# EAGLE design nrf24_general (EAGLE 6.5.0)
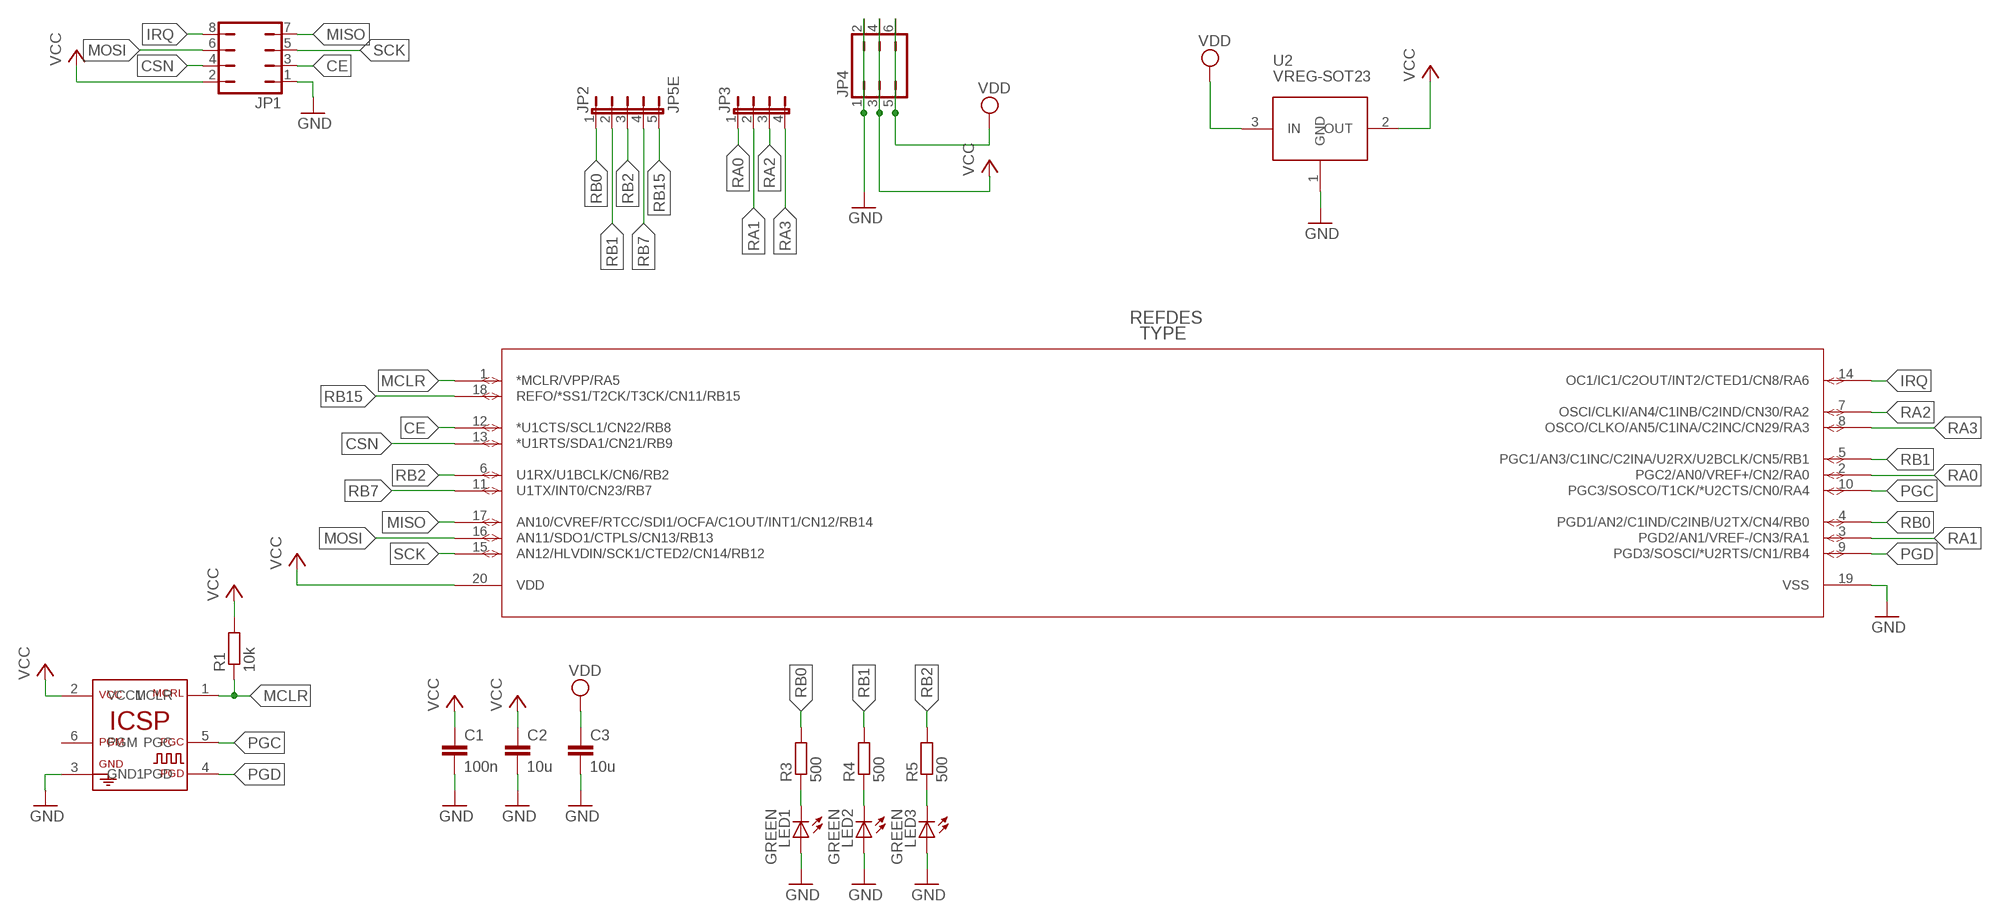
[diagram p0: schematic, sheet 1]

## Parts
C1  100n  C-EUC0603  [C0603]
C2  10u  C-EUC0805  [C0805]
C3  10u  C-EUC0805  [C0805]
ICSP  PICKIT3  [PICKIT3]
JP1  JP4Q  [JP4Q]
JP2  JP5E  [JP5]
JP3  JP4E  [JP4]
JP4  JP3Q  [JP3Q]
LED1  GREEN  LEDCHIP-LED0603  [CHIP-LED0603]
LED2  GREEN  LEDCHIP-LED0603  [CHIP-LED0603]
LED3  GREEN  LEDCHIP-LED0603  [CHIP-LED0603]
R1  10k  R-EU_R0603  [R0603]
R3  500  R-EU_R0603  [R0603]
R4  500  R-EU_R0603  [R0603]
R5  500  R-EU_R0603  [R0603]
U2  VREG-SOT23  [SOT-23]
U3  PIC24F16KA101-X_  [SSOP20_MC]

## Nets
CE: JP1.3 U3.12(*U1CTS/SCL1/CN22/RB8)
CSN: JP1.4 U3.13(*U1RTS/SDA1/CN21/RB9)
GND: C1.2 C2.2 C3.2 ICSP.3(GND1) JP1.1 JP4.1 JP4.2 LED1.A LED2.A LED3.A U2.1(GND) U3.19(VSS)
IRQ: JP1.8 U3.14(OC1/IC1/C2OUT/INT2/CTED1/CN8/RA6)
MCLR: ICSP.1(MCLR) R1.1 U3.1(*MCLR/VPP/RA5)
MISO: JP1.7 U3.17(AN10/CVREF/RTCC/SDI1/OCFA/C1OUT/INT1/CN12/RB14)
MOSI: JP1.6 U3.16(AN11/SDO1/CTPLS/CN13/RB13)
N$2: LED1.C R3.1
N$3: LED2.C R4.1
N$4: LED3.C R5.1
PGC: ICSP.5(PGC) U3.10(PGC3/SOSCO/T1CK/*U2CTS/CN0/RA4)
PGD: ICSP.4(PGD) U3.9(PGD3/SOSCI/*U2RTS/CN1/RB4)
RA0: JP3.1 U3.2(PGC2/AN0/VREF+/CN2/RA0)
RA1: JP3.2 U3.3(PGD2/AN1/VREF-/CN3/RA1)
RA2: JP3.3 U3.7(OSCI/CLKI/AN4/C1INB/C2IND/CN30/RA2)
RA3: JP3.4 U3.8(OSCO/CLKO/AN5/C1INA/C2INC/CN29/RA3)
RB0: JP2.1 R3.2 U3.4(PGD1/AN2/C1IND/C2INB/U2TX/CN4/RB0)
RB1: JP2.2 R4.2 U3.5(PGC1/AN3/C1INC/C2INA/U2RX/U2BCLK/CN5/RB1)
RB2: JP2.3 R5.2 U3.6(U1RX/U1BCLK/CN6/RB2)
RB7: JP2.4 U3.11(U1TX/INT0/CN23/RB7)
RB15: JP2.5 U3.18(REFO/*SS1/T2CK/T3CK/CN11/RB15)
SCK: JP1.5 U3.15(AN12/HLVDIN/SCK1/CTED2/CN14/RB12)
VCC: C1.1 C2.1 ICSP.2(VCC1) JP1.2 JP4.3 JP4.4 R1.2 U2.2(OUT) U3.20(VDD)
VDD: C3.1 JP4.5 JP4.6 U2.3(IN)

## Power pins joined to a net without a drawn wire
PGM: ICSP.6(PGM)

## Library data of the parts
C1-C3 = rcl:C-EU: CAPACITOR, European symbol
ICSP = other:PICKIT3
JP1 = jumper_own:JP4Q: JUMPER
JP2 = jumper_own:JP5E
JP3 = jumper_own:JP4E: JUMPER
JP4 = jumper:JP3Q: JUMPER
LED1-LED3 = led:LED: LED
R1 R3-R5 = rcl:R-EU_: RESISTOR, European symbol
U2 = other:VREG-SOT23
U3 = microchip:PIC24F16KA101-X_

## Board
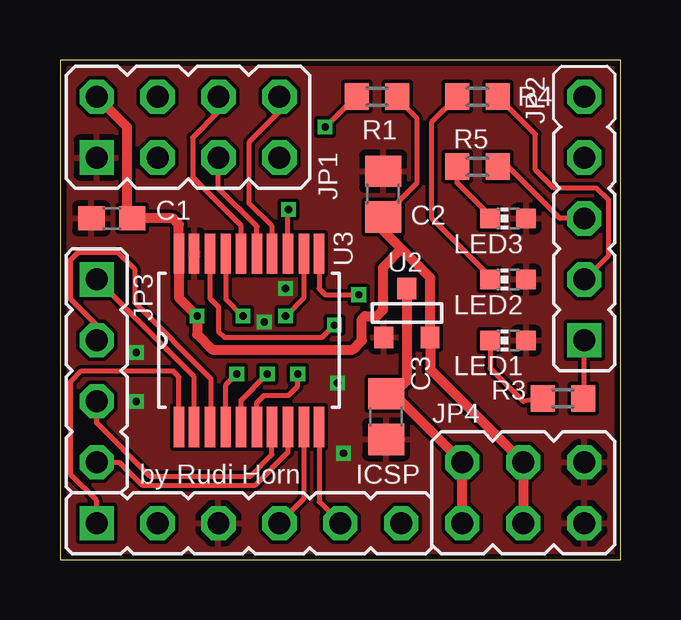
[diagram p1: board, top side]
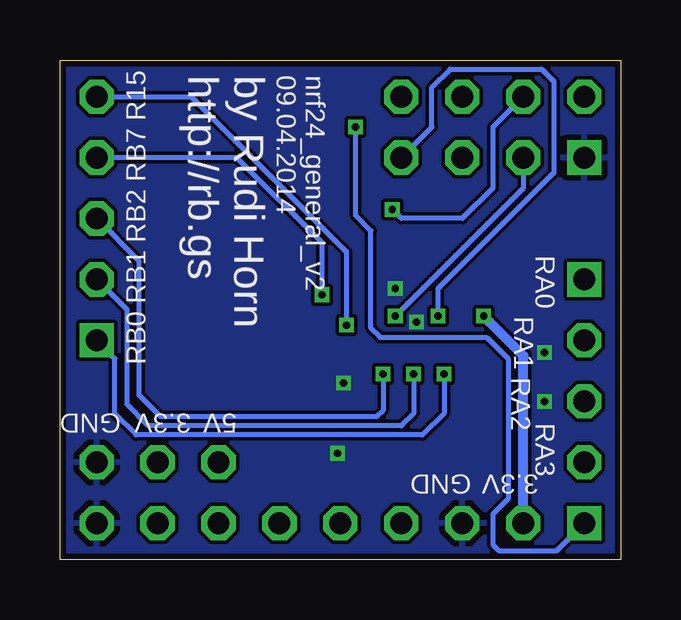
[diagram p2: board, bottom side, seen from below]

Size 23.37 x 20.83 mm. Coordinates in mm from the lower left corner, seen from the top.
Outline: 0,0 23.37,0 23.37,20.83 0,20.83 0,0
Copper layers (1*16): Top 0.035mm / dielectric 1.5mm / Bottom 0.035mm
Design rules "Elecrow_2-layer_eagle_rule": minimum track width 6mil, minimum drill 12mil, track to track 6mil, track to pad 6mil, pad to pad 6mil, via to via 6mil, smd to smd 0mil, copper to edge 10mil, drill to drill 10mil, minimum pad ring 10mil, minimum via ring 6mil, stop-mask expansion 2mil, vias tented up to drill 100mil, thermal gap 10mil

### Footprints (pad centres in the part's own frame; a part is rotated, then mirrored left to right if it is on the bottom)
C0603 = smd 1.1 x 1: 1 -0.85,0; 2 0.85,0
C0805 = smd 1.3 x 1.5: 1 -0.95,0; 2 0.95,0
PICKIT3 = drill 0.914 square: 1 -3.81,0 | drill 0.914 octagon: 2 -1.27,0; 3 1.27,0; 4 3.81,0; 5 6.35,0; 6 8.89,0
JP4Q = drill 0.914 square: 1 -3.81,-1.27 | drill 0.914 octagon: 2 -3.81,1.27; 3 -1.27,-1.27; 4 -1.27,1.27; 5 1.27,-1.27; 6 1.27,1.27; 7 3.81,-1.27; 8 3.81,1.27
JP5 = drill 0.914 square: 1 -3.81,0 | drill 0.914 octagon: 2 -1.27,0; 3 1.27,0; 4 3.81,0; 5 6.35,0
JP4 = drill 0.914 square: 1 -3.81,0 | drill 0.914 octagon: 2 -1.27,0; 3 1.27,0; 4 3.81,0
JP3Q = drill 0.914 octagon: 1 -2.54,-1.27; 2 -2.54,1.27; 3 0,-1.27; 4 0,1.27; 5 2.54,-1.27; 6 2.54,1.27
CHIP-LED0603 = smd 0.8 x 0.8: A 0,-0.75; C 0,0.75
R0603 = smd 1 x 1.1: 1 -0.85,0; 2 0.85,0
SOT-23 = smd 0.787 x 0.889: 1 0.991,1.016; 2 -0.94,1.016; 3 0.025,-1.016
SSOP20_MC = smd 1.676 x 0.432: 1 -3.607,2.921; 2 -3.607,2.286; 3 -3.607,1.626; 4 -3.607,0.965; 5 -3.607,0.33; 6 -3.607,-0.33; 7 -3.607,-0.965; 8 -3.607,-1.626; 9 -3.607,-2.286; 10 -3.607,-2.921; 11 3.607,-2.921; 12 3.607,-2.286; 13 3.607,-1.626; 14 3.607,-0.965; 15 3.607,-0.33; 16 3.607,0.33; 17 3.607,0.965; 18 3.607,1.626; 19 3.607,2.286; 20 3.607,2.921

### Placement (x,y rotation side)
C1  2.16,14.22 180 top
C2  13.46,15.24 90 top
C3  13.59,5.97 270 top
ICSP  5.33,1.52 0 top
JP1  5.33,18.03 0 top
JP2  21.84,12.95 90 top
JP3  1.52,7.87 270 top
JP4  19.3,2.79 180 top
LED1  18.67,9.14 90 top
LED2  18.67,11.68 90 top
LED3  18.67,14.22 90 top
R1  13.21,19.3 0 top
R3  20.96,6.73 0 top
R4  17.4,19.3 0 top
R5  17.4,16.38 0 top
U2  14.48,10.29 180 top
U3  7.87,9.14 90 top

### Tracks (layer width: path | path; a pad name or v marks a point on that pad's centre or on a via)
CE  (via drill 0.3 pad 0.2)
  Top 0.203: U3.12 10.16,10.92 v9.4,10.16
  Bottom 0.203: JP1.3 4.06,15.49 v9.4,10.16
CSN  (via drill 0.3)
  Top 0.203: U3.13 9.5,14.45 v9.53,14.61
  Bottom 0.203: JP1.4 5.33,18.03 5.33,15.49 6.6,14.22 9.14,14.22 v9.53,14.61
GND  (via drill 0.3)
  other vias: 3.17,6.6 3.17,8.64 9.4,11.3 8.51,9.91 11.56,7.37 11.81,4.45
  pour Top: 0,0 23.37,0 23.37,20.83 0,20.83
  pour Bottom: 23.37,0 0,0 0,20.83 23.37,20.83
IRQ
  Top 0.203: JP1.8 9.14,18.67 7.87,17.4 7.87,14.86 8.84,13.89 U3.14
MCLR  (via drill 0.3)
  Top 0.203: ICSP.1 1.52,2.48 0.45,3.56 0.45,7.43 0.89,7.87 4.7,7.87 4.95,7.62 U3.1 | R1.1 12.32,19.3 v11.05,18.03
  Bottom 0.203: ICSP.1 2.67,0.38 5.08,0.38 5.33,0.64 5.33,1.91 4.7,2.54 4.7,8.38 5.59,9.27 10.03,9.27 10.41,9.65 10.41,13.72 11.05,14.35 v11.05,18.03
MISO  (via drill 0.3)
  Top 0.203: v7.62,10.16 6.91,10.87 U3.17
  Bottom 0.203: JP1.7 7.87,18.03 7.87,19.69 7.11,20.45 3.3,20.45 2.79,19.94 2.79,16.13 7.62,11.3 v7.62,10.16
MOSI
  Top 0.203: JP1.6 6.6,18.67 5.53,17.59 5.53,15.94 7.54,13.92 U3.16
N$2
  Top 0.203: R3.1 19.3,6.6 17.92,7.99 LED1.C
N$3
  Top 0.203: 17.92,11.8 15.49,14.22 15.49,18.25 R4.1
  Top 0.406: LED2.C 17.92,11.8
N$4
  Top 0.203: 17.92,14.34 16.55,15.71 R5.1
  Top 0.406: LED3.C 17.92,14.34
PGC
  Top 0.203: U3.10 10.79,2.41 ICSP.5
PGD
  Top 0.203: U3.9 10.16,2.54 ICSP.4
RA0
  Top 0.203: U3.2 5.59,7.62 JP3.1
RA1
  Top 0.203: JP3.2 1.52,9.78 0.45,10.86 0.45,12.51 0.76,12.83 2.41,12.83 3.11,12.13 3.11,10.73 6.29,7.56 6.29,5.57 U3.3
RA2
  Top 0.203: U3.7 8.83,5.53 8.83,4.38 7.94,3.49 3.75,3.49 1.52,5.71 JP3.3
RA3
  Top 0.203: JP3.4 2.48,4.06 3.43,3.11 8.13,3.11 9.5,4.48 U3.8
RB0  (via drill 0.3)
  Top 0.203: U3.4 6.91,7.29 v7.37,7.75 | R3.2 21.84,6.77 JP2.1
  Bottom 0.203: v7.37,7.75 7.37,6.1 8.25,5.21 20.19,5.21 21.08,6.1 21.08,8.38 JP2.1
RB1  (via drill 0.3)
  Top 0.203: U3.5 7.54,6.65 v8.64,7.75 | JP2.2 22.86,12.7 22.86,14.99 22.35,15.49 20.57,15.49 19.81,16.26 19.81,17.74 R4.2
  Bottom 0.203: v8.64,7.75 8.64,6.1 9.14,5.59 19.69,5.59 20.57,6.48 20.57,10.41 JP2.2
RB2  (via drill 0.3)
  Top 0.203: U3.6 8.2,6.55 8.51,6.86 9.53,6.86 9.91,7.24 v9.91,7.75 | JP2.3 20.83,14.22 18.67,16.38 R5.2
  Bottom 0.203: v9.91,7.75 9.91,6.22 10.16,5.97 19.18,5.97 20.07,6.86 20.07,12.45 JP2.3
RB7  (via drill 0.3)
  Top 0.203: U3.11 10.79,11.3 11.05,11.05 v12.45,11.05
  Bottom 0.203: v12.45,11.05 12.45,13.21 16,16.76 JP2.4
RB15  (via drill 0.3 pad 0.2)
  Top 0.203: U3.18 6.25,10.9 6.6,10.54 6.6,9.53 6.86,9.27 10.92,9.27 v11.43,9.78
  Bottom 0.203: JP2.5 17.91,19.3 11.43,12.83 v11.43,9.78
SCK
  Top 0.203: U3.15 8.2,13.89 6.6,15.49 JP1.5
VCC  (via drill 0.3)
  Top 0.203: 2.79,14.44 C1.1 | 13.46,13.72 C2.1 14.86,15.69 14.86,18.42 14.06,19.22 R1.2
  Top 0.406: C1.1 4.7,14.22 4.95,13.97 U3.20 4.95,10.92 v5.71,10.16 5.71,9.4 6.35,8.76 12.19,8.76 12.57,9.14 12.57,10.03 12.7,10.16 13.21,10.16 13.46,10.41 13.46,12.19 14.22,12.95 | 2.79,14.44 2.79,18.03 JP1.2 | JP4.4 JP4.3 15.42,7.95 U2.2 15.42,11.76 14.22,12.95 | 14.22,12.95 13.46,13.72
  Bottom 0.406: ICSP.2 4.06,8.51 v5.71,10.16
VDD
  Top 0.406: JP4.6 JP4.5 13.91,6.92 | U2.3 14.45,7.46 13.91,6.92 | 13.91,6.92 C3.1

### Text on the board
tNames: by Rudi Horn
bNames: nrf24_general_v2 / 09.04.2014 | by Rudi Horn / http://rb.gs | R15 | RB7 | RB2 | RA0 | RA1 | RB1 | RB0 | RA2 | 5V | 3.3V | GND | RA3 | 3.3V | GND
